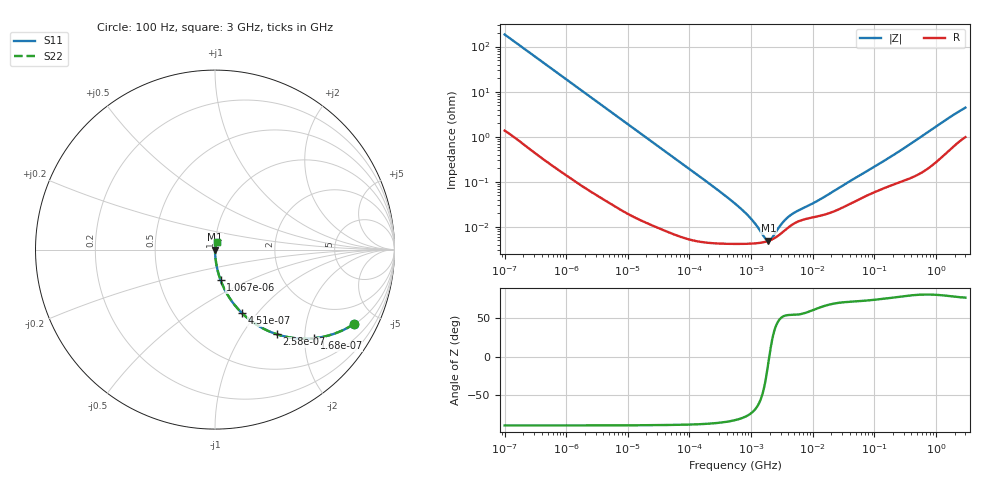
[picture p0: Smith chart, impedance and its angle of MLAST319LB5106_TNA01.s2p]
! MLAST319LB5106_TNA01  S-PARAMETER MODEL  ( Standard Model )
! Model Generated by TAIYO YUDEN Corporation (http://www.ty-top.com)
! Version 1.0
! TAIYO YUDEN Control No. 220601
! Copyright(c) 2009 TAIYO YUDEN CO.,LTD. All Rights Reserved.
! Product Description (link to TY-COMPAS)
! https://ds.yuden.co.jp/TYCOMPAS/or/detail?pn=MLAST319LB5106KTNA01&u=M
! Products Name : Multilayer Ceramic Capacitors
! Characteristics :
!  Capacitance : 10 [uF] , Rated Voltage : 25 [V] , TCC : X5R
!  Case Size : 3.2 x 1.6 / 0.126 x 0.063 [mm/inch] , Thickness : 0.85 / 0.033 [mm/inch]
!  (Conditions: Temperature = 25 [degC] , DC Bias Voltage = 0 [V])
! External Node Assignments :
!  1  o---| |---o  2
! GND o---------o GND
! Frequency Range : 100Hz  -  3GHz  [ 401 STEP ]
# MHZ S RI R 50
! Freq[MHz].  S11 Real  S11 Imag  S21 Real  S21 Imag  S12 Real  S12 Imag  S22 Real  S22 Imag
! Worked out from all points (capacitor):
!   401 points, 100 Hz to 3 GHz, reference 50 ohm
!   read as one part in series: C = 8.56 uF near 109 Hz
!   lowest |Z| = 4.92 mohm at 1.908 MHz (marker M1)
!   series resonance near 1.971 MHz, so ESL is about 760 pH
!   S11 on the Smith chart (normalised r, x): 100 Hz: 1.03, -3.71; 168 Hz: 1.02, -2.22; 258 Hz: 1.01, -1.45; 451 Hz: 1.01, -0.83; 1.067 kHz: 1.00, -0.35; 3 GHz: 1.02, +0.09
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0.0001  0.7733 -0.415  0.2267 0.415  0.2267 0.415  0.7733 -0.415
0.000168  0.5519 -0.4936  0.4481 0.4936  0.4481 0.4936  0.5519 -0.4936
0.000258  0.3448 -0.4717  0.6552 0.4717  0.6552 0.4717  0.3448 -0.4717
0.000451  0.1485 -0.352  0.8515 0.352  0.8515 0.352  0.1485 -0.352
0.000664  0.0752 -0.2602  0.9248 0.2602  0.9248 0.2602  0.0752 -0.2602
0.001067  0.0312 -0.1702  0.9688 0.1702  0.9688 0.1702  0.0312 -0.1702
0.001788  0.0117 -0.1039  0.9883 0.1039  0.9883 0.1039  0.0117 -0.1039
0.005476  0.0015 -0.0345  0.9985 0.0345  0.9985 0.0345  0.0015 -0.0345
0.031977  0.000128 -0.00597  0.9999 0.00597  0.9999 0.00597  0.000128 -0.00597
0.221826  4.45e-05 -0.000858  1 0.000858  1 0.000858  4.45e-05 -0.000858
0.547723  4.19e-05 -0.000326  1 0.000326  1 0.000326  4.19e-05 -0.000326
0.842342  4.21e-05 -0.000189  1 0.000189  1 0.000189  4.21e-05 -0.000189
1.240863  4.33e-05 -9.51e-05  1 9.51e-05  1 9.51e-05  4.33e-05 -9.51e-05
1.411895  4.43e-05 -6.76e-05  1 6.76e-05  1 6.76e-05  4.43e-05 -6.76e-05
1.908323  4.88e-05 -6.42e-06  1 6.42e-06  1 6.42e-06  4.88e-05 -6.42e-06
2.81117  6.51e-05 7.07e-05  0.9999 -7.07e-05  0.9999 -7.07e-05  6.51e-05 7.07e-05
3.79959  9.1e-05 0.000126  0.9999 -0.000126  0.9999 -0.000126  9.1e-05 0.000126
4.711951  0.000113 0.000159  0.9999 -0.000159  0.9999 -0.000159  0.000113 0.000159
9.794414  0.000161 0.000284  0.9998 -0.000284  0.9998 -0.000284  0.000161 0.000284
175.1444  0.000811 0.00335  0.9992 -0.00335  0.9992 -0.00335  0.000811 0.00335
1506.733  0.00504 0.024  0.995 -0.024  0.995 -0.024  0.00504 0.024
3000  0.0115 0.0422  0.9885 -0.0422  0.9885 -0.0422  0.0115 0.0422
